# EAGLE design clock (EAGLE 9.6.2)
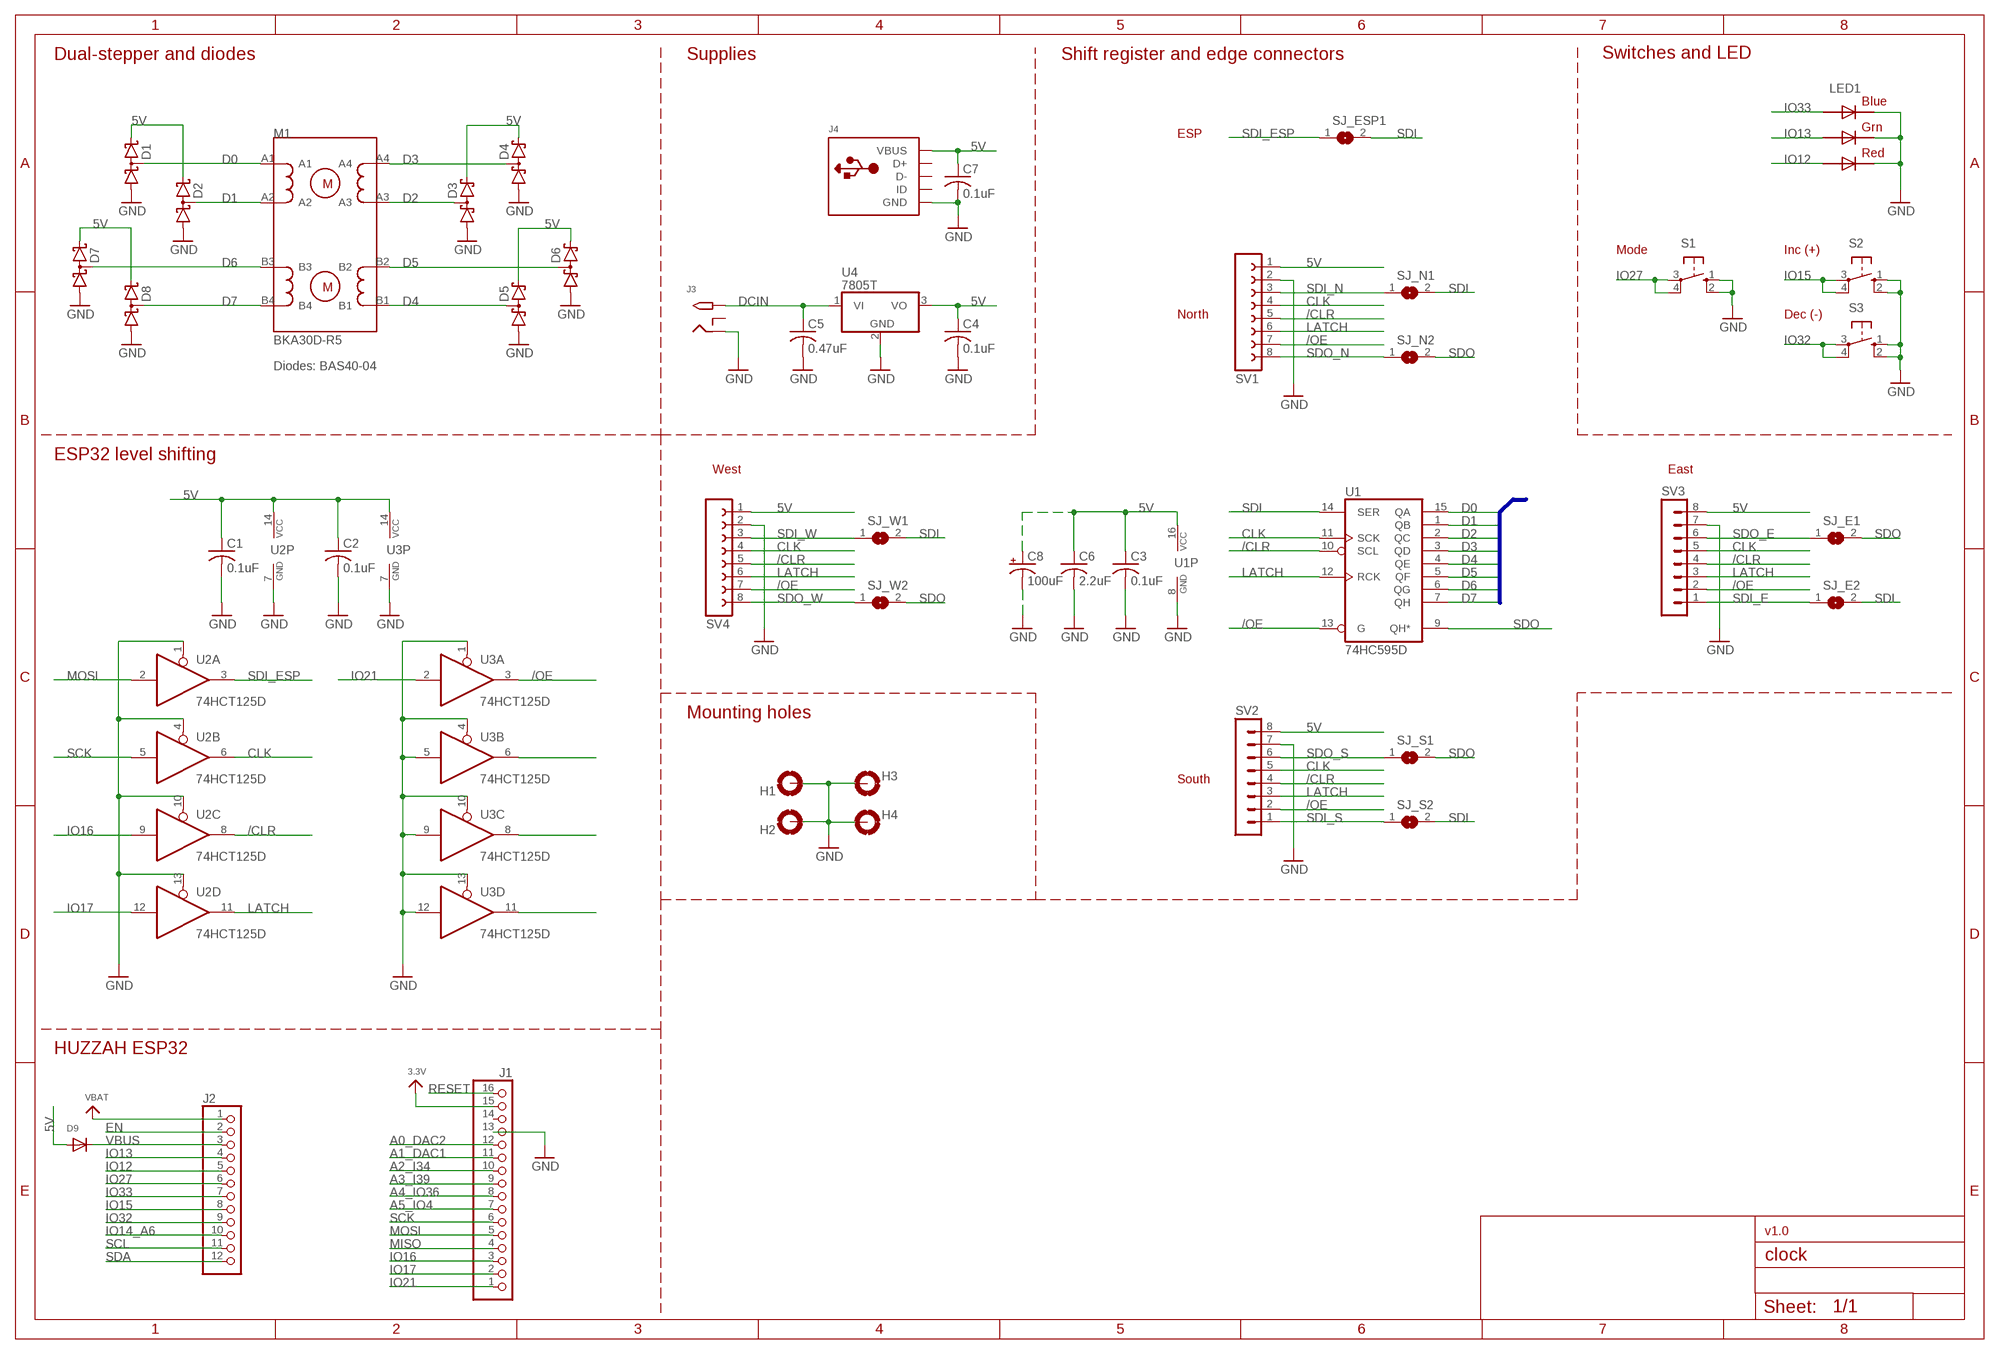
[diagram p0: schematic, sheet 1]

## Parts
C1  0.1uF  C-USC0805K  [C0805K]
C2  0.1uF  C-USC0805K  [C0805K]
C3  0.1uF  C-USC0805K  [C0805K]
C4  0.1uF  C-USC0805K  [C0805K]
C5  0.47uF  C-USC0805K  [C0805K]
C6  2.2uF  C-USC0805K  [C0805K]
C7  0.1uF  C-USC0805K  [C0805K]
C8  100uF  CPOL-USE3.5-8  [E3,5-8]
D1  BAS40-04  [SOT23]
D2  BAS40-04  [SOT23]
D3  BAS40-04  [SOT23]
D4  BAS40-04  [SOT23]
D5  BAS40-04  [SOT23]
D6  BAS40-04  [SOT23]
D7  BAS40-04  [SOT23]
D8  BAS40-04  [SOT23]
D9  DIODEDO-1N4148  [DO-1N4148]
H1  MOUNT-PAD-ROUND4.3  [4,3-PAD]
H2  MOUNT-PAD-ROUND4.3  [4,3-PAD]
H3  MOUNT-PAD-ROUND4.3  [4,3-PAD]
H4  MOUNT-PAD-ROUND4.3  [4,3-PAD]
J1  HEADER-1X16_MIN  [1X16_ROUND_MIN]
J2  HEADER-1X12_MIN  [1X12_ROUND_MIN]
J3  2.1MMJACKTHM  [PJ-102A]
J4  USBMINIB  [USB-MINIB]
LED1  RGBLED5050  [RGBLED5050]
M1  BKA30D-R5  [BKA30D-R5]
S1  10-XX  [B3F-10XX]
S2  10-XX  [B3F-10XX]
S3  10-XX  [B3F-10XX]
SJ_E1  SJ  [SJ]
SJ_E2  SJ  [SJ]
SJ_ESP1  SJ  [SJ]
SJ_N1  SJ  [SJ]
SJ_N2  SJ  [SJ]
SJ_S1  SJ  [SJ]
SJ_S2  SJ  [SJ]
SJ_W1  SJ  [SJ]
SJ_W2  SJ  [SJ]
SV1  FE08W  [FE08W]
SV2  MA08-1W  [MA08-1W]
SV3  MA08-1W  [MA08-1W]
SV4  FE08W  [FE08W]
U1  74HC595D  [SO16]
U2  74HCT125D  [SO14]
U3  74HCT125D  [SO14]
U4  7805T  [TO220H]

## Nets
3.3V: J1.15
5V: C1.1 C2.1 C3.1 C4.1 C6.1 C7.1 C8.+ D1.2(C2) D2.2(C2) D3.2(C2) D4.2(C2) D5.2(C2) D6.2(C2) D7.2(C2) D8.2(C2) D9.A J4.VBUS SV1.1 SV2.8 SV3.8 SV4.1 U1.16(VCC) U2.14(P:VCC) U3.14(P:VCC) U4.3(VO)
/CLR: SV1.5 SV2.4 SV3.4 SV4.5 U1.10(SCL) U2.8(C:O)
/OE: SV1.7 SV2.2 SV3.2 SV4.7 U1.13(G) U3.3(A:O)
A0_DAC2: J1.12
A1_DAC1: J1.11
A2_I34: J1.10
A3_I39: J1.9
A4_IO36: J1.8
A5_IO4: J1.7
CLK: SV1.4 SV2.5 SV3.5 SV4.4 U1.11(SCK) U2.6(B:O)
D0: D1.3(C1A2) M1.A1 U1.15(QA)
D1: D2.3(C1A2) M1.A2 U1.1(QB)
D2: D3.3(C1A2) M1.A3 U1.2(QC)
D3: D4.3(C1A2) M1.A4 U1.3(QD)
D4: D5.3(C1A2) M1.B1 U1.4(QE)
D5: D6.3(C1A2) M1.B2 U1.5(QF)
D6: D7.3(C1A2) M1.B3 U1.6(QG)
D7: D8.3(C1A2) M1.B4 U1.7(QH)
DCIN: C5.1 J3.TIP U4.1(VI)
EN: J2.2
GND: C1.2 C2.2 C3.2 C4.2 C5.2 C6.2 C7.2 C8.- D1.1(A1) D2.1(A1) D3.1(A1) D4.1(A1) D5.1(A1) D6.1(A1) D7.1(A1) D8.1(A1) H1.B4,3(MOUNT) H2.B4,3(MOUNT) H3.B4,3(MOUNT) H4.B4,3(MOUNT) J1.13 J3.RING J4.GND LED1.4(BLUE_C) LED1.5(RED_C) LED1.6(GREEN_C) S1.1(S) S1.2(S1) S2.1(S) S2.2(S1) S3.1(S) S3.2(S1) SV1.2 SV2.7 SV3.7 SV4.2 U1.8(GND) U2.1(A:OE) U2.4(B:OE) U2.7(P:GND) U2.10(C:OE) U2.13(D:OE) U3.1(A:OE) U3.4(B:OE) U3.5(B:I) U3.7(P:GND) U3.9(C:I) U3.10(C:OE) U3.12(D:I) U3.13(D:OE) U4.2(GND)
IO12: J2.5 LED1.2(RED_A)
IO13: J2.4 LED1.1(GREEN_A)
IO14_A6: J2.10
IO15: J2.8 S2.3(P) S2.4(P1)
IO16: J1.3 U2.9(C:I)
IO17: J1.2 U2.12(D:I)
IO21: J1.1 U3.2(A:I)
IO27: J2.6 S1.3(P) S1.4(P1)
IO32: J2.9 S3.3(P) S3.4(P1)
IO33: J2.7 LED1.3(BLUE_A)
LATCH: SV1.6 SV2.3 SV3.3 SV4.6 U1.12(RCK) U2.11(D:O)
MISO: J1.4
MOSI: J1.5 U2.2(A:I)
N$1: U3.11(D:O)
N$2: U3.8(C:O)
N$3: U3.6(B:O)
RESET: J1.16
SCK: J1.6 U2.5(B:I)
SCL: J2.11
SDA: J2.12
SDI: SJ_E2.2 SJ_ESP1.2 SJ_N1.2 SJ_S2.2 SJ_W1.2 U1.14(SER)
SDI_E: SJ_E2.1 SV3.1
SDI_ESP: SJ_ESP1.1 U2.3(A:O)
SDI_N: SJ_N1.1 SV1.3
SDI_S: SJ_S2.1 SV2.1
SDI_W: SJ_W1.1 SV4.3
SDO: SJ_E1.2 SJ_N2.2 SJ_S1.2 SJ_W2.2 U1.9(QH*)
SDO_E: SJ_E1.1 SV3.6
SDO_N: SJ_N2.1 SV1.8
SDO_S: SJ_S1.1 SV2.6
SDO_W: SJ_W2.1 SV4.8
VBAT: J2.1
VBUS: D9.C J2.3
Unconnected: J1.14 J3.RING_SW J4.D+ J4.D- J4.ID

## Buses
D[0..7]

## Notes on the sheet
- Dual-stepper and diodes | Supplies | Shift register and edge connectors | Switches and LED
- ESP
- Mode | Inc (+)
- North | Dec (-)
- Diodes: BAS40-04
- ESP32 level shifting
- West | East
- Mounting holes
- South
- HUZZAH ESP32
- v1.0

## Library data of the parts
C1-C7 = rcl:C-US: CAPACITOR, American symbol; SPICEPREFIX: C
C8 = rcl:CPOL-US: POLARIZED CAPACITOR, American symbol; SPICEPREFIX: C
D1-D8 = diode:BAS40-04: Silicon Schottky Diodes General-purpose diode for high-speed switching
D9 = adafruit:DIODE: Diode
H1-H4 = holes:MOUNT-PAD-ROUND: MOUNTING PAD, round
J1 = microbuilder:HEADER-1X16: PIN HEADER
J2 = microbuilder:HEADER-1X12
J3 = adafruit:2.1MMJACK: 2.1mm x 5.5mm THM DC jack with internal switch. Digikey part #PJ-102A, 4UCON part #05537 2.1mm x 5.5mm SMT DC jack with internal switch. Digikey part #PJ-002A-SMT, 4UCON part #03267 By microbuilder.eu & adafruit.com
J4 = adafruit:USB: USB Connectors USBMINIB - Surface Mount Female Mini-B USB Connector 4UConnector: 06564 By microbuilder.eu Thru-hole RA Female Mini-B USB Connector 4UConnector: 18732 By ladyada.net
LED1 = adafruit:RGBLED: For 5050 RGB LEDs, the order of the LEDs may vary from one manufacturer to another!
M1 = my_components:BKA30D-R5
S1-S3 = switch-omron:10-XX: OMRON SWITCH; MPN: B3F-1000; OC_FARNELL: 176432; OC_NEWARK: 36M3542
SJ_E1 SJ_E2 SJ_ESP1 SJ_N1 SJ_N2 SJ_S1 SJ_S2 SJ_W1 SJ_W2 = jumper:SJ: SMD solder JUMPER
SV1 SV4 = con-lsta:FE08W: FEMALE HEADER; OC_FARNELL: unknown; OC_NEWARK: unknown
SV2 SV3 = con-lstb:MA08-1W: PIN HEADER; OC_FARNELL: unknown; OC_NEWARK: unknown
U1 = 74xx-eu:74*595: 8-bit SHIFT REGISTER, output latch
U2 U3 = 74xx-eu:74*125: Quad bus BUFFER, 3-state
U4 = adafruit:78*: Positive VOLTAGE REGULATOR Added bigger pads to the TO-92 package

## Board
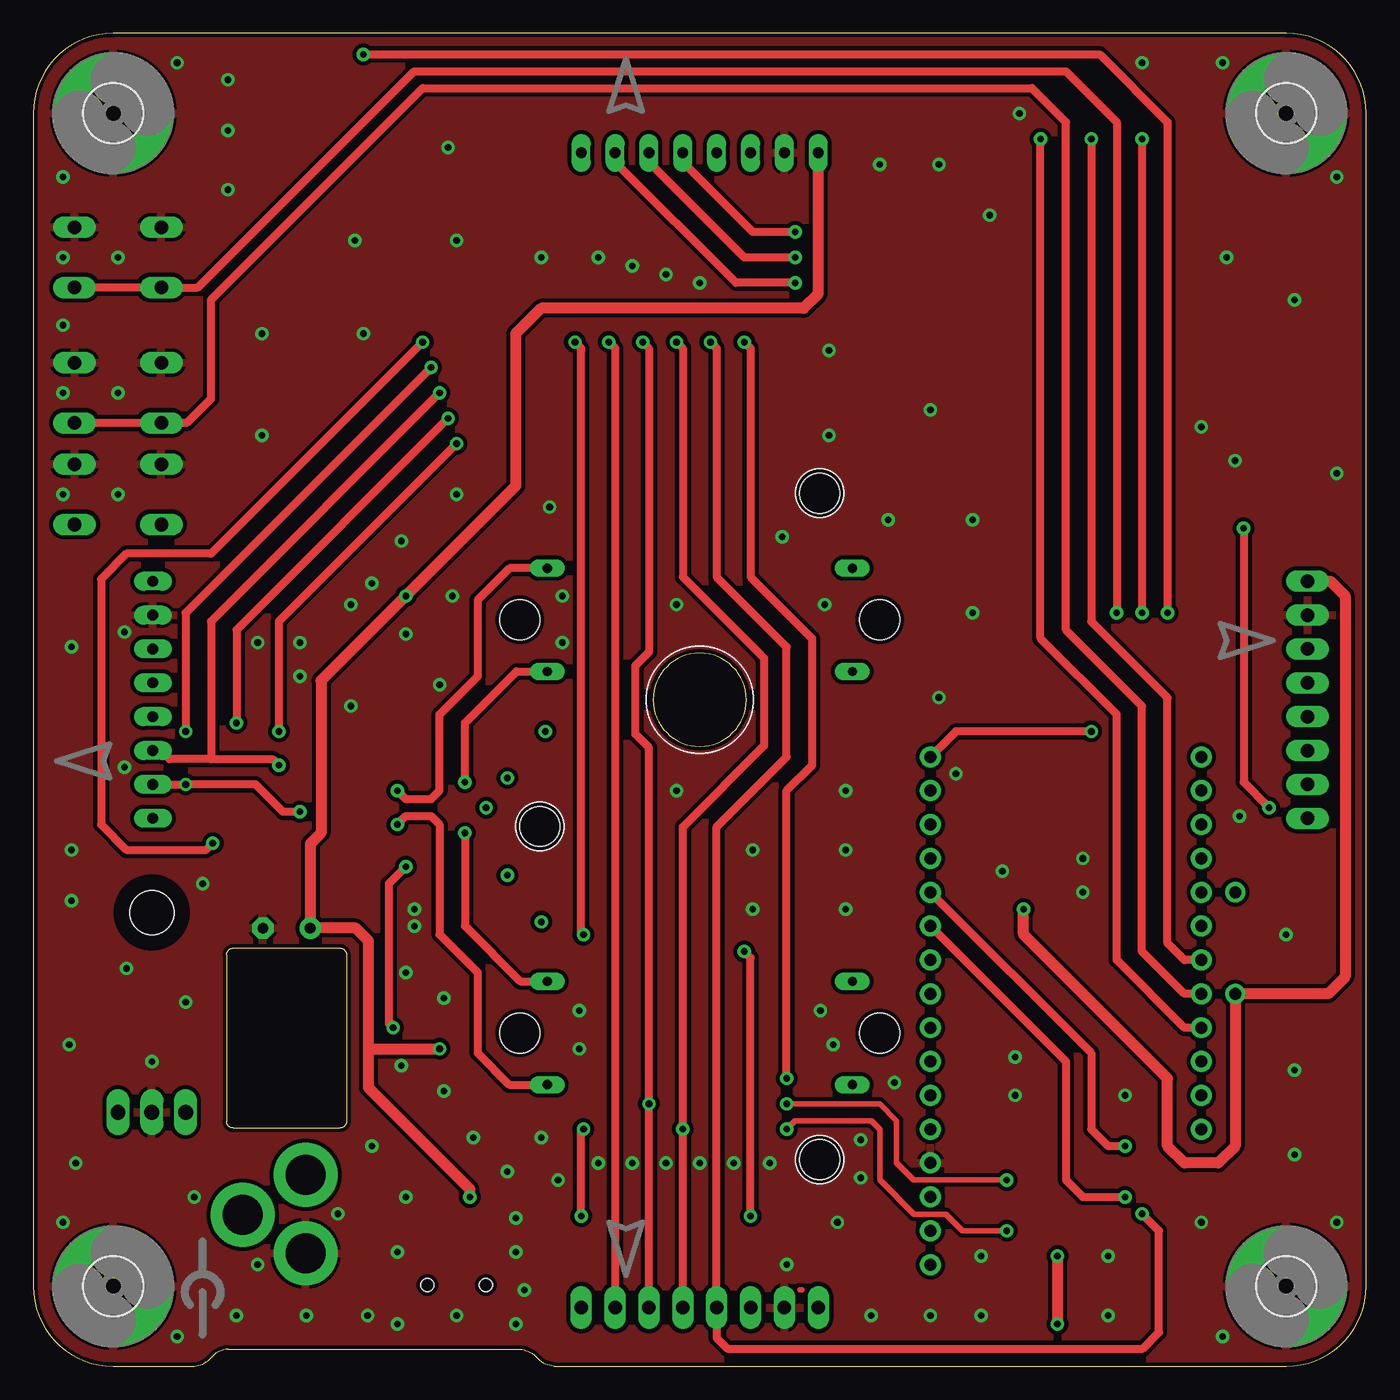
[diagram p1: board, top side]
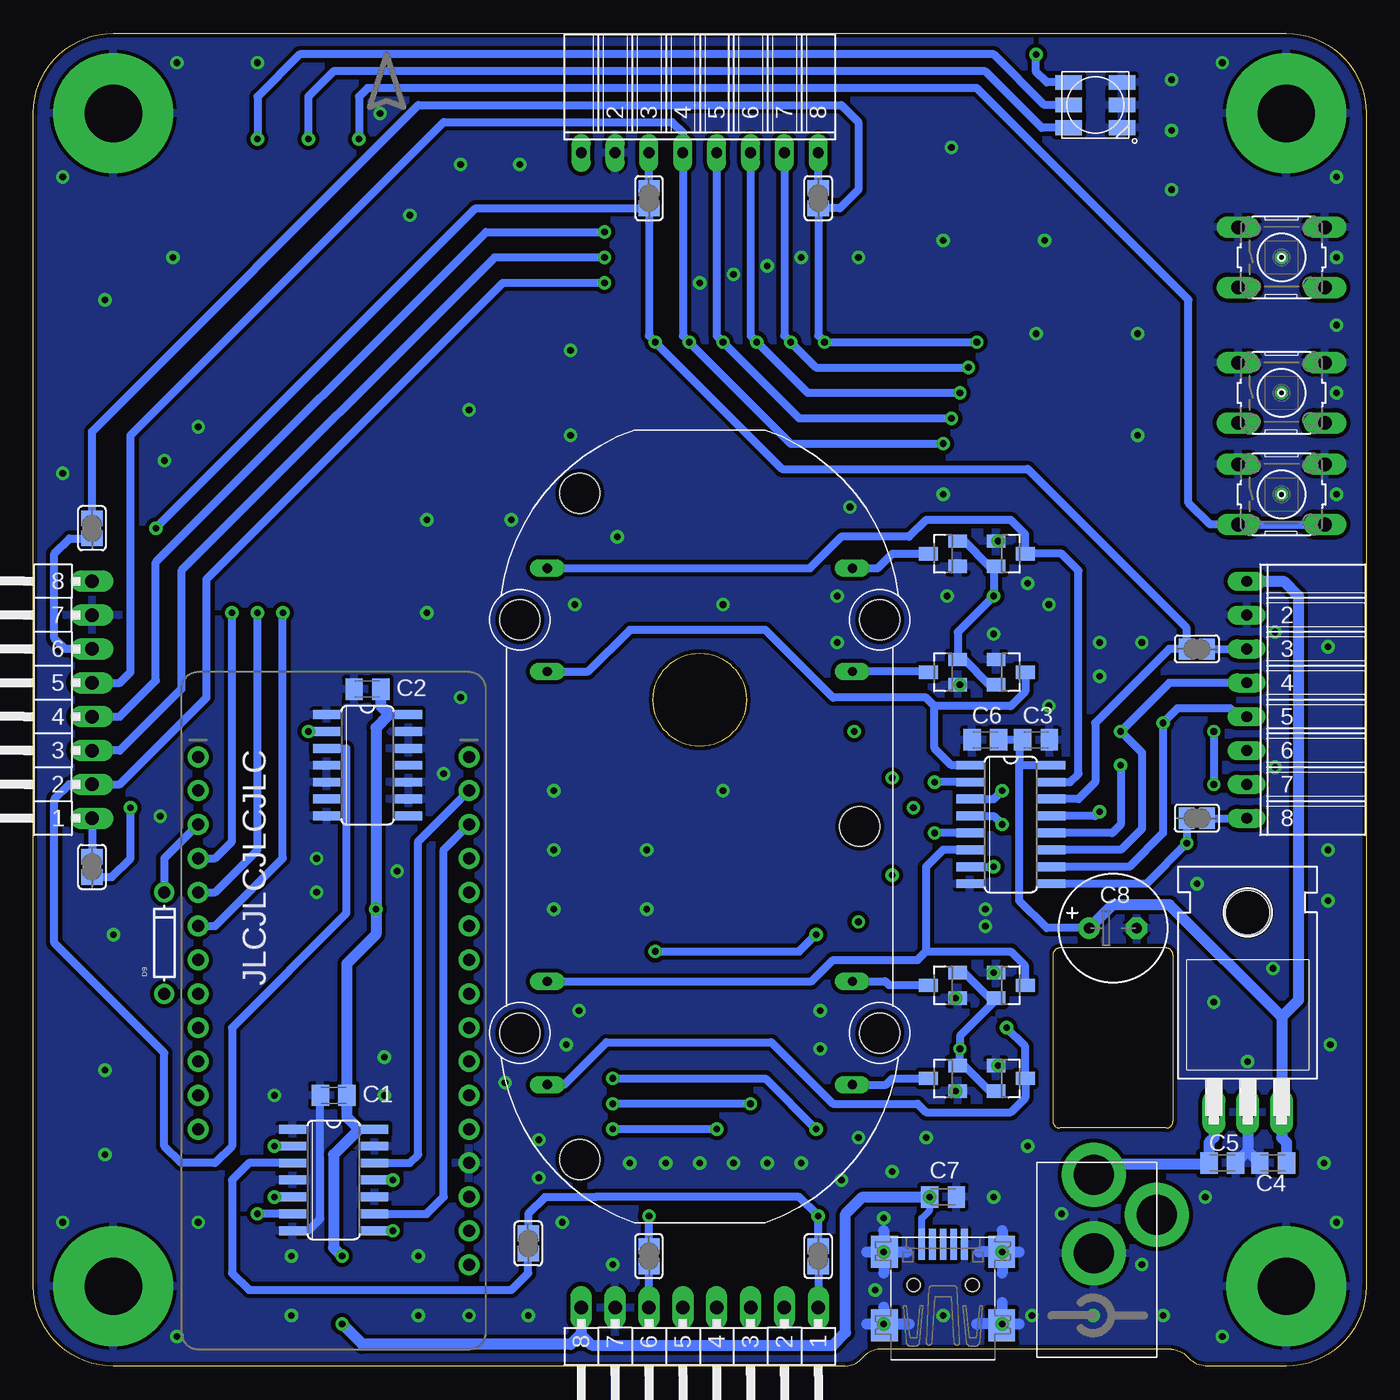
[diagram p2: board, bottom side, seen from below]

Size 100 x 100 mm. Coordinates in mm from the lower left corner, seen from the top.
Outline: 6,0 12.06,0 arc45 13.34,0.64 arc-45 14.61,1.27 36.51,1.27 arc-45 37.78,0.64 arc45 39.05,0 94,0 arc90 100,6 100,94 arc90 94,100 6,100 arc90 0,94 0,6 arc90 6,0
Outline: 14.5,30.86 14.5,18.36 arc90 15,17.86 23,17.86 arc90 23.5,18.36 23.5,30.86 arc90 23,31.36 15,31.36 arc90 14.5,30.86
Copper layers (1*16): Top 0.035559375mm / dielectric 1.6mm / Bottom 0.035559375mm
Design rules "jlcpcb2layer": minimum track width 5mil, minimum drill 8mil, track to track 5mil, track to pad 5mil, pad to pad 20mil, via to via 10mil, smd to smd 5mil, copper to edge 8mil, drill to drill 20mil, minimum pad ring 12mil, minimum via ring 5mil, stop-mask expansion 2.5mil, vias tented up to drill 20mil, thermal gap 10mil

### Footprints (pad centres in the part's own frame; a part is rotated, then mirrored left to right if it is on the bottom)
C0805K = smd 1.3 x 1.6: 1 -1,0; 2 1,0
E3,5-8 = drill 0.813 pad 1.6: + -1.778,0 | drill 0.813 pad 1.6 octagon: - 1.778,0
SOT23 = smd 1 x 1.4: 1 -0.95,-1.1; 2 0.95,-1.1; 3 0,1.1
DO-1N4148 = drill 0.9: A -3.81,0; C 3.81,0
4,3-PAD = drill 4.3 pad 9: B4,3 0,0
1X16_ROUND_MIN = drill 0.9 pad 1.575: 1 -19.05,0; 2 -16.51,0; 3 -13.97,0; 4 -11.43,0; 5 -8.89,0; 6 -6.35,0; 7 -3.81,0; 8 -1.27,0; 9 1.27,0; 10 3.81,0; 11 6.35,0; 12 8.89,0; 13 11.43,0; 14 13.97,0; 15 16.51,0; 16 19.05,0
1X12_ROUND_MIN = drill 0.9 pad 1.575: 1 -13.97,0; 2 -11.43,0; 3 -8.89,0; 4 -6.35,0; 5 -3.81,0; 6 -1.27,0; 7 1.27,0; 8 3.81,0; 9 6.35,0; 10 8.89,0; 11 11.43,0; 12 13.97,0
PJ-102A = drill 3 pad 4.8: RING 0.1,-3.39; RING_SW -4.6,-6.29; TIP 0.1,-9.29
USB-MINIB = smd 0.5 x 2.308: D+ 0,4.064; D- -0.8,4.064; GND 1.6,4.064; ID 0.8,4.064; VBUS -1.6,4.064 | smd 2 x 2.4: GND1 -4.4,-2; GND2 -4.4,3.5; GND3 4.4,3.5; GND4 4.4,-2 | hole 1: -2.2,1; 2.2,1
RGBLED5050 = smd 2 x 1.1: 1 -2,1.7; 2 -2,0; 3 -2,-1.7; 4 2,-1.7; 5 2,0; 6 2,1.7
BKA30D-R5 = drill 0.7 long: A1 19.375,11.45; A2 11.625,11.45; A3 11.625,-11.45; A4 19.375,-11.45; B1 -19.375,-11.45; B2 -11.625,-11.45; B3 -11.625,11.45; B4 -19.375,11.45 | hole 3: -15.5,13.5; -15.5,-13.5; 15.5,-13.5; 15.5,13.5; -25,9; 25,9; 0,-12
B3F-10XX = drill 1.016 long: 1 -3.251,2.261; 2 3.251,2.261; 3 -3.251,-2.261; 4 3.251,-2.261
SJ = smd 1.168 x 1.6: 1 -0.762,0; 2 0.762,0
FE08W = drill 0.813 long: 1 -8.89,0; 2 -6.35,0; 3 -3.81,0; 4 -1.27,0; 5 1.27,0; 6 3.81,0; 7 6.35,0; 8 8.89,0
MA08-1W = drill 1.016 long: 1 -8.89,0; 2 -6.35,0; 3 -3.81,0; 4 -1.27,0; 5 1.27,0; 6 3.81,0; 7 6.35,0; 8 8.89,0
SO16 = smd 0.66 x 2.032: 1 -4.445,-3.073; 2 -3.175,-3.073; 3 -1.905,-3.073; 4 -0.635,-3.073; 5 0.635,-3.073; 6 1.905,-3.073; 7 3.175,-3.073; 8 4.445,-3.073; 9 4.445,3.073; 10 3.175,3.073; 11 1.905,3.073; 12 0.635,3.073; 13 -0.635,3.073; 14 -1.905,3.073; 15 -3.175,3.073; 16 -4.445,3.073
SO14 = smd 0.66 x 2.032: 1 -3.81,-3.073; 2 -2.54,-3.073; 3 -1.27,-3.073; 4 0,-3.073; 5 1.27,-3.073; 6 2.54,-3.073; 7 3.81,-3.073; 8 3.81,3.073; 9 2.54,3.073; 10 1.27,3.073; 11 0,3.073; 12 -1.27,3.073; 13 -2.54,3.073; 14 -3.81,3.073
TO220H = drill 1.118 long: 1 -2.54,-10.16; 2 0,-10.16; 3 2.54,-10.16 | hole 3.302: 0,4.826

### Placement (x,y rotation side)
C1  77.47,20.32 180 bottom
C2  74.93,50.8 180 bottom
C3  24.77,46.99 0 bottom
C4  6.99,15.24 180 bottom
C5  10.79,15.24 0 bottom
C6  28.57,46.99 180 bottom
C7  31.75,12.7 0 bottom
C8  19,32.87 0 bottom
D1  26.67,60.96 270 bottom
D2  26.67,52.07 270 bottom
D3  31.75,52.07 90 bottom
D4  31.75,60.96 90 bottom
D5  31.75,21.59 90 bottom
D6  31.75,28.57 90 bottom
D7  26.67,28.57 270 bottom
D8  26.67,21.59 270 bottom
D9  90.17,31.75 90 bottom
H1  6,94 0 top
H2  94,94 0 top
H3  6,6 0 top
H4  94,6 0 top
J1  67.31,26.67 270 bottom
J2  87.63,31.75 270 bottom
J3  20.32,5.08 180 bottom
J4  31.75,5.08 0 bottom
LED1  20.32,94.61 0 bottom
M1  50,40.5 90 bottom
S1  6.35,83.19 0 bottom
S2  6.35,73.03 0 bottom
S3  6.35,65.41 0 bottom
SJ_E1  95.6,62.87 90 bottom
SJ_E2  95.6,37.47 270 bottom
SJ_ESP1  62.87,9.21 90 bottom
SJ_N1  53.81,87.63 270 bottom
SJ_N2  41.11,87.63 270 bottom
SJ_S1  53.81,8.26 90 bottom
SJ_S2  41.11,8.26 90 bottom
SJ_W1  12.7,53.81 180 bottom
SJ_W2  12.7,41.11 180 bottom
SV1  50,91.04 0 bottom
SV2  50,4.4 180 bottom
SV3  95.6,50 90 bottom
SV4  8.96,50 270 bottom
U1  26.67,40.64 270 bottom
U2  77.47,13.97 270 bottom
U3  74.93,45.09 270 bottom
U4  8.89,29.21 0 bottom

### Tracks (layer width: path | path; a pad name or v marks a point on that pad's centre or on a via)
5V  (via drill 0.5 pad 1)
  Top 0.813: C7.1 32.75,13.29 25.14,20.9 25.14,23.81 | SV1.1 58.89,80.48 57.78,79.38 38.1,79.38 36.2,77.47 36.2,66.04 v27.94,57.78 21.59,51.44 21.59,40.01 20.78,39.19 C8.+ 24.18,32.87 25.14,31.91 25.14,23.81 | v76.83,8.26 v76.83,3.17 | SV3.8 97.32,58.89 98.42,57.78 98.42,29.21 97.16,27.94 D9.A 90.17,16.51 88.9,15.24 86.36,15.24 85.09,16.51 85.09,21.59 74.3,32.38 v74.3,34.29 | 25.14,23.81 v30.48,23.81
  Bottom 0.508: J4.VBUS 33.35,11.1 32.75,11.7 C7.1
  Bottom 0.61: 73.3,48.9 U3.14 | U2.14 75.56,17.78 | D6.2 30.16,29.52 28.26,27.62 D7.2 27.77,27.48 30.48,24.77 v30.48,23.81 30.48,22.71 D5.2 30.16,22.54 28.26,20.64 D8.2 | D2.2 28.26,51.12 30.16,53.02 D3.2 30.65,55.08 v27.94,57.78 27.94,59.84 D1.2 28.26,60.01 30.16,61.91 D4.2 | 26.04,45.09 26.04,46.72 C3.1 C6.1 | 26.04,45.09 26.04,34.92 23.98,32.87 C8.+ | U1.16 26.04,45.09
  Bottom 0.813: C2.1 73.93,49.53 73.3,48.9 74.3,47.9 v74.3,34.29 74.3,32.38 76.47,30.21 C1.1 76.47,18.68 75.56,17.78 77.47,15.88 77.47,8.89 v76.83,8.26 | C4.1 5.99,16.78 6.35,17.14 U4.3 6.35,26.19 | 6.35,26.19 14.77,34.61 19.04,34.61 C8.+ | v76.83,3.17 75.3,1.64 59.69,1.64 58.89,2.44 SV2.8 58.89,2.38 58.1,1.59 40.01,1.59 39.05,2.54 39.05,11.43 37.78,12.7 C7.1 | SV4.1 6.18,58.89 5.08,57.78 5.08,27.46 6.35,26.19
  other vias: 32.75,12.7
/CLR  (via drill 0.5 pad 1)
  Top 0.406: v73.03,10.16 69.7,10.16 68.46,11.4 66.06,11.4 63.5,13.97 63.5,17.78 62.87,18.41 57.15,18.41 v56.52,17.78
  Top 0.61: v31.11,71.12 15.24,55.24 v15.24,48.26 | SV1.5 48.73,90.33 53.98,85.09 v57.15,85.09 | SV2.4 v48.73,17.78 48.73,40.48 54.82,46.57 54.82,53.12 54.61,53.33 54.61,53.34 48.73,59.22 48.73,76.36 v48.26,76.83
  Bottom 0.61: SV4.5 9.6,48.73 10.23,49.37 14.13,49.37 v15.24,48.26 15.24,40.01 17.78,37.47 U1.10 | SV1.5 48.73,77.31 v48.26,76.83 42.55,71.12 v31.11,71.12 | SV3.4 93.51,48.73 90.81,51.44 90.81,60.33 66.04,85.09 v57.15,85.09 | U2.8 v73.03,10.16 | v48.73,17.78 v56.52,17.78
/OE  (via drill 0.5 pad 1)
  Top 0.61: v20,41.59 18.73,41.59 16.68,43.65 v11.43,43.65 SV4.7 | v11.43,47.62 11.43,56.52 v29.84,74.93 | v57.15,81.28 52.7,81.28 43.65,90.33 SV1.7 | v43.18,76.83 43.65,76.36 SV2.2
  Bottom 0.61: v20,41.59 20.32,41.27 U1.13 | SV1.7 43.65,77.31 v43.18,76.83 41.27,74.93 v29.84,74.93 | v11.43,47.62 v11.43,43.65 | v57.15,81.28 64.77,81.28 87,59.05 87,50.16 93.51,43.65 SV3.2 97.32,43.65 98.42,42.55 98.42,31.75 90.17,23.5 90.17,16.51 88.9,15.24 86.36,15.24 85.09,16.51 85.09,25.4 76.52,33.97 76.52,46.35 U3.3
CLK  (via drill 0.5 pad 1)
  Top 0.61: v31.75,69.22 18.41,55.88 v18.41,47.62 | v83.19,11.43 84.45,10.16 84.45,2.54 83.24,1.32 52.07,1.32 51.27,2.12 SV2.5 51.27,40.48 56.52,45.72 56.52,53.98 51.27,59.22 51.27,76.36 v50.8,76.83
  Bottom 0.61: SV4.4 14.77,51.27 v18.41,47.62 16.83,46.04 16.83,40.32 18.41,38.73 U1.11 | v31.75,69.22 43.18,69.22 v50.8,76.83 51.27,77.31 SV1.4 51.27,92.55 52.07,93.34 69.22,93.34 92.71,69.85 92.71,52.07 93.51,51.27 SV3.5 | U2.6 v83.19,11.43
D0
  Bottom 0.61: M1.A1 41.73,59.88 39.37,62.23 34.29,62.23 33.02,63.5 26.67,63.5 25.57,62.4 D1.3 22.86,60.96 21.59,59.69 21.59,44.45 22.23,43.81 U1.15
D1
  Bottom 0.61: D2.3 25.57,50.63 26.67,49.53 32.38,49.53 | 32.38,49.53 33.02,50.16 40.01,50.16 45.09,55.24 55.24,55.24 58.37,52.12 M1.A2 | U1.1 31.11,45.09 32.38,46.35 32.38,49.53
D2  (via drill 0.5 pad 1)
  Top 0.61: v32.38,43.81 32.38,48.26 36.25,52.12 M1.A3
  Bottom 0.61: D3.3 32.91,52.12 M1.A3 | U1.2 v32.38,43.81
D3  (via drill 0.5 pad 1)
  Top 0.61: M1.A4 35.74,59.88 33.34,57.47 33.34,51.75 30.48,48.9 30.48,43.18 29.84,42.55 27.94,42.55 v27.3,43.18
  Bottom 0.61: D4.3 35.56,60.96 36.65,59.88 M1.A4 | U1.3 27.94,42.55 v27.3,43.18
D4  (via drill 0.5 pad 1)
  Top 0.61: M1.B1 35.71,21.12 33.34,23.5 33.34,29.53 30.48,32.38 30.48,40.64 29.84,41.27 27.94,41.27 v27.3,40.64
  Bottom 0.61: M1.B1 36.02,21.12 35.56,21.59 D5.3 | U1.4 27.94,41.27 v27.3,40.64
D5  (via drill 0.5 pad 1)
  Top 0.61: v32.38,40.01 32.38,33.02 36.53,28.88 M1.B2
  Bottom 0.61: D6.3 35.77,28.57 36.07,28.88 M1.B2 | U1.5 v32.38,40.01
D6
  Bottom 0.61: D7.3 25.57,30.02 26.67,31.11 31.11,31.11 33.02,31.11 | M1.B3 41.61,28.88 40.01,30.48 33.66,30.48 33.02,31.11 | U1.6 31.75,38.73 33.02,37.47 33.02,31.11
D7  (via drill 0.5 pad 1)
  Top 0.61: v27.94,37.47 26.67,36.2 26.67,25.72 v26.99,25.4
  Bottom 0.61: M1.B4 60.18,21.12 57.01,24.3 44.62,24.3 40.01,19.68 33.66,19.68 33.02,19.05 26.67,19.05 25.57,20.15 D8.3 25.57,23.98 v26.99,25.4 | U1.7 v27.94,37.47
DCIN
  Bottom 0.813: U4.1 11.43,17.14 11.79,16.78 C5.1 11.86,15.17 19.62,15.17 J3.TIP
GND  (via drill 0.5 pad 1)
  Bottom 0.61: U2.7 79.38,10.16 78.47,11.06 C1.2 | D8.1 v27.62,22.54 | D1.1 v27.62,61.91 | D3.1 v30.48,51.12 | D7.1 v27.94,29.53 | D5.1 v30.8,20.64 | D6.1 v30.8,27.62
  Bottom 0.813: 8.89,16.14 C4.2 | U4.2 8.89,16.14 | 8.89,16.14 C5.2 | v27.3,3.17 26.04,3.17 | v27.3,3.17 27.3,4.76 | 27.3,10.16 v27.3,8.57 | v27.3,8.57 27.3,6.99 | v27.3,8.57 26.04,8.57 | 36.2,10.16 v36.2,8.57 | v36.2,8.57 36.2,6.99 | 37.47,8.57 v36.2,8.57 | 36.2,4.45 v36.2,3.17 | 37.47,3.17 v36.2,3.17 | v27.3,3.17 29.21,3.17 | v36.2,3.17 34.29,3.17 | v27.3,8.57 29.05,8.57 | v36.2,8.57 34.45,8.57
  other vias: 64.14,63.5 59.69,69.85 67.31,71.75 70.48,63.5 70.48,56.52 59.69,76.2 60.96,43.18 60.96,38.73 60.96,34.29 53.98,38.73 48.26,43.18 53.98,34.29 63.5,90.17 67.94,90.17 71.75,86.36 87.63,70.48 90.17,67.94 89.53,83.19 94.61,80.01 31.11,91.44 31.75,84.45 24.13,84.45 24.77,77.47 17.14,77.47 17.14,69.85 6.35,65.41 6.35,73.03 6.35,83.19 14.61,88.27 14.61,92.71 14.61,96.52 31.75,65.41 38.73,64.45 31.43,57.78 23.81,57.15 25.4,58.74 38.1,17.14 40.96,23.81 40.96,26.67 2.86,34.92 11.43,27.3 6.99,29.84 12.7,36.2 3.17,15.24 2.7,24.13 8.89,22.86 15.24,3.81 25.08,3.81 2.86,38.73 2.86,53.98 27.94,54.93 23.81,49.53 28.57,33.02 28.57,34.29 89.22,97.79 97.79,89.22 10.79,97.79 2.22,89.22 2.22,10.79 10.79,2.22 89.22,2.22 97.79,10.79 2.22,83.19 2.22,78.11 2.22,73.03 2.22,65.41 83.19,97.79 72.71,37.15 69.22,44.45 78.74,38.1 78.74,35.56 73.66,23.18 93.98,32.38 94.61,22.23 97.79,66.99 87.63,10.79 94.61,15.88 81.92,20.32 73.66,20.32 20.48,3.81 25.4,16.51 27.94,12.7 36.83,5.71 36.2,11.11 44.93,15.24 50.01,15.24 47.47,15.24 52.55,15.24 56.52,7.62 60.33,10.79 55.24,15.24 62.87,3.81 67.31,3.81 71.12,3.81 71.12,8.26 80.64,3.81 80.64,8.26 39.37,13.97 42.39,15.24 59.05,26.67 60.01,24.13 33.02,17.14 35.56,14.61 12.06,12.7 16.83,7.62 22.86,11.43 39.69,54.29 39.69,57.78 48.26,57.15 59.37,57.15 56.2,62.23 38.1,83.19 42.39,83.19 44.93,82.55 47.47,81.92 50.01,81.28 16.83,54.29 20,54.29 20,51.75 62.07,16.99 62.07,14.13 64.61,21.27 67.94,50.16 73.98,93.98 31.75,3.81 6.83,44.93 6.83,55.09 90.49,41.27
  pour Top (isolate 0.305): 0,100.33 0,0 100.33,0 100.33,100.33
  pour Bottom (isolate 0.305): 0,100.33 0,0 100.33,0 100.33,100.33
IO12  (via drill 0.5 pad 1)
  Top 0.61: v83.19,92.08 v83.19,56.52
  Bottom 0.61: J2.5 86.36,35.56 83.19,38.73 v83.19,56.52 | LED1.2 24.13,94.61 27.94,98.42 80.01,98.42 83.19,95.25 v83.19,92.08
IO13  (via drill 0.5 pad 1)
  Top 0.61: v24.77,98.42 80.01,98.42 85.09,93.34 v85.09,56.52
  Bottom 0.61: J2.4 86.36,38.1 85.09,39.37 v85.09,56.52 | LED1.1 23.97,96.31 24.77,97.11 v24.77,98.42
IO15
  Top 0.61: J2.8 86.36,27.94 83.19,31.11 83.19,49.53 77.47,55.24 77.47,93.34 74.93,95.89 29.21,95.89 13.34,80.01 13.34,72.59 11.51,70.76 S2.3 S2.4
IO16
  Bottom 0.61: U2.9 70.48,11.43 69.22,12.7 69.22,38.73 J1.3
IO17
  Bottom 0.61: U2.12 71.75,15.24 71.12,15.88 71.12,39.37 J1.2
IO21  (via drill 0.5 pad 1)
  Top 0.61: v79.38,47.62 69.22,47.62 J1.1
  Bottom 0.61: U3.2 v79.38,47.62
IO27  (via drill 0.5 pad 1)
  Top 0.61: v81.28,56.52 81.28,93.34 77.47,97.16 28.57,97.16 12.34,80.92 S1.3 S1.4
  Bottom 0.61: J2.6 86.36,33.02 81.28,38.1 v81.28,56.52
IO32  (via drill 0.5 pad 1)
  Top 0.61: v75.56,92.08 75.56,54.61 81.28,48.9 81.28,30.48 86.36,25.4 J2.9
  Bottom 0.61: v75.56,92.08 75.56,95.25 74.93,95.89 29.21,95.89 13.34,80.01 13.34,64.77 11.71,63.14 S3.3 S3.4
IO33  (via drill 0.5 pad 1)
  Top 0.61: J2.7 86.36,30.48 85.09,31.75 85.09,50.16 79.38,55.88 v79.38,92.08
  Bottom 0.61: LED1.3 24.34,92.92 28.57,97.16 77.47,97.16 79.38,95.25 v79.38,92.08
LATCH  (via drill 0.5 pad 1)
  Top 0.406: v73.03,13.97 66.04,13.97 64.77,15.24 64.77,18.41 63.5,19.68 v56.52,19.68
  Top 0.61: 13.34,45.55 10.23,45.55 9.6,46.19 SV4.6 | v30.48,73.03 13.34,55.88 13.34,45.55 | v18.41,45.09 17.95,45.55 13.34,45.55 | SV1.6 46.19,90.33 53.34,83.19 v57.15,83.19 | SV2.3 v46.19,19.68 46.19,46.41 45.18,47.42 45.18,52.55 46.19,53.56 46.19,76.36 v45.72,76.83
  Bottom 0.61: v18.41,45.09 18.41,40.64 19.05,40.01 U1.12 | SV1.6 46.19,77.31 v45.72,76.83 41.91,73.03 v30.48,73.03 | v57.15,83.19 65.41,83.19 88.9,59.69 88.9,50.8 93.51,46.19 SV3.3 | U2.11 v73.03,13.97 | v46.19,19.68 v56.52,19.68
MOSI  (via drill 0.5 pad 1)
  Top 0.61: v81.92,16.51 80.64,16.51 79.38,17.78 79.38,23.5 J1.5
  Bottom 0.61: v81.92,16.51 U2.2
N$4
  Top 0.406: 57.66,5.71 57.53,5.71
N$10  (via drill 0.5 pad 1)
  other vias: 38.42,47.62
N$11  (via drill 0.5 pad 1)
  other vias: 35.56,44.13
N$12  (via drill 0.5 pad 1)
  other vias: 33.97,41.91
N$13  (via drill 0.5 pad 1)
  other vias: 35.56,36.83
N$14  (via drill 0.5 pad 1)
  other vias: 38.1,33.34
SCK  (via drill 0.5 pad 1)
  Top 0.61: v81.92,12.7 78.74,12.7 77.47,13.97 77.47,22.86 J1.6
  Bottom 0.61: U2.5 v81.92,12.7
SDI  (via drill 0.5 pad 1)
  Top 0.61: v90.81,62.87 90.81,43.81 v92.71,41.91 | v41.27,17.78 41.11,17.61 v41.11,11.27 | v56.52,21.59 56.52,43.18 58.42,45.09 58.42,54.61 53.81,59.22 53.81,76.36 v53.34,76.83
  Bottom 0.61: U1.14 21.59,42.55 20.32,43.81 20.32,48.26 14.77,53.81 SJ_W1.2 13.46,55.37 25.4,67.31 43.81,67.31 v53.34,76.83 53.81,77.31 SJ_N1.2 66.8,86.87 v90.81,62.87 | SJ_E2.2 94.11,36.7 92.71,38.1 v92.71,41.91 | SJ_S2.2 v41.11,11.27 42.55,12.7 57.81,12.7 57.83,12.68 61.62,12.68 62.87,11.43 SJ_ESP1.2 | v41.27,17.78 45.09,21.59 v56.52,21.59
SDI_E
  Bottom 0.61: SV3.1 SJ_E2.1
SDI_ESP
  Bottom 0.61: U2.3 83.82,15.24 85.09,13.97 85.09,6.99 83.82,5.71 64.14,5.71 62.87,6.99 SJ_ESP1.1
SDI_N
  Bottom 0.61: SJ_N1.1 SV1.3
SDI_S
  Bottom 0.61: SJ_S2.1 SV2.1
SDI_W
  Bottom 0.61: SJ_W1.1 SV4.3
SDO  (via drill 0.5 pad 1)
  Top 0.61: v29.21,76.83 13.34,60.96 6.99,60.96 5.08,59.05 5.08,40.64 6.99,38.73 12.95,38.73 v13.46,39.24 | v53.34,31.11 53.81,30.64 v53.81,11.27 | v41.27,32.38 41.11,32.55 41.11,76.2 41.11,76.36 v40.64,76.83
  Bottom 0.61: v29.21,76.83 v40.64,76.83 41.11,77.31 SJ_N2.2 39.5,86.87 38.1,88.27 38.1,93.34 39.37,94.61 71.12,94.61 95.6,70.14 SJ_E1.2 | SJ_W2.2 v13.46,39.24 16.51,36.2 U1.9 | SJ_S1.2 v53.81,11.27 | v53.34,31.11 42.55,31.11 v41.27,32.38
SDO_E
  Bottom 0.61: SV3.6 97.62,53.81 98.42,54.61 98.42,60.96 97.28,62.1 SJ_E1.1
SDO_N
  Bottom 0.61: SJ_N2.1 SV1.8
SDO_S
  Bottom 0.61: SV2.6 SJ_S1.1
SDO_W
  Bottom 0.61: SJ_W2.1 SV4.8
VBUS
  Bottom 0.61: J2.3 90.17,38.1 D9.C

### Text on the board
bPlace: JLCJLCJLCJLC
tStop: ClockClock24
tDocu: North | v1.0 | Mode | (+) | (-) | East | West | - | South | + | 12V | DC | USB
bDocu: North | Status | < | IN | OUT | > | > | M | + | - | OUT | > | < | IN | > | HUZZAH32 | HCT125 | HC595 | OUT | > | < | IN | > | 7805 | HCT125 | > | > | > | OUT | 12VDC | USB | ESP / IN | IN | - | + | <

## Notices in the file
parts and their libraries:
microbuilder: This work is placed in the public domain, and may be freely used for commercial and non-commercial work with the following conditions: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
